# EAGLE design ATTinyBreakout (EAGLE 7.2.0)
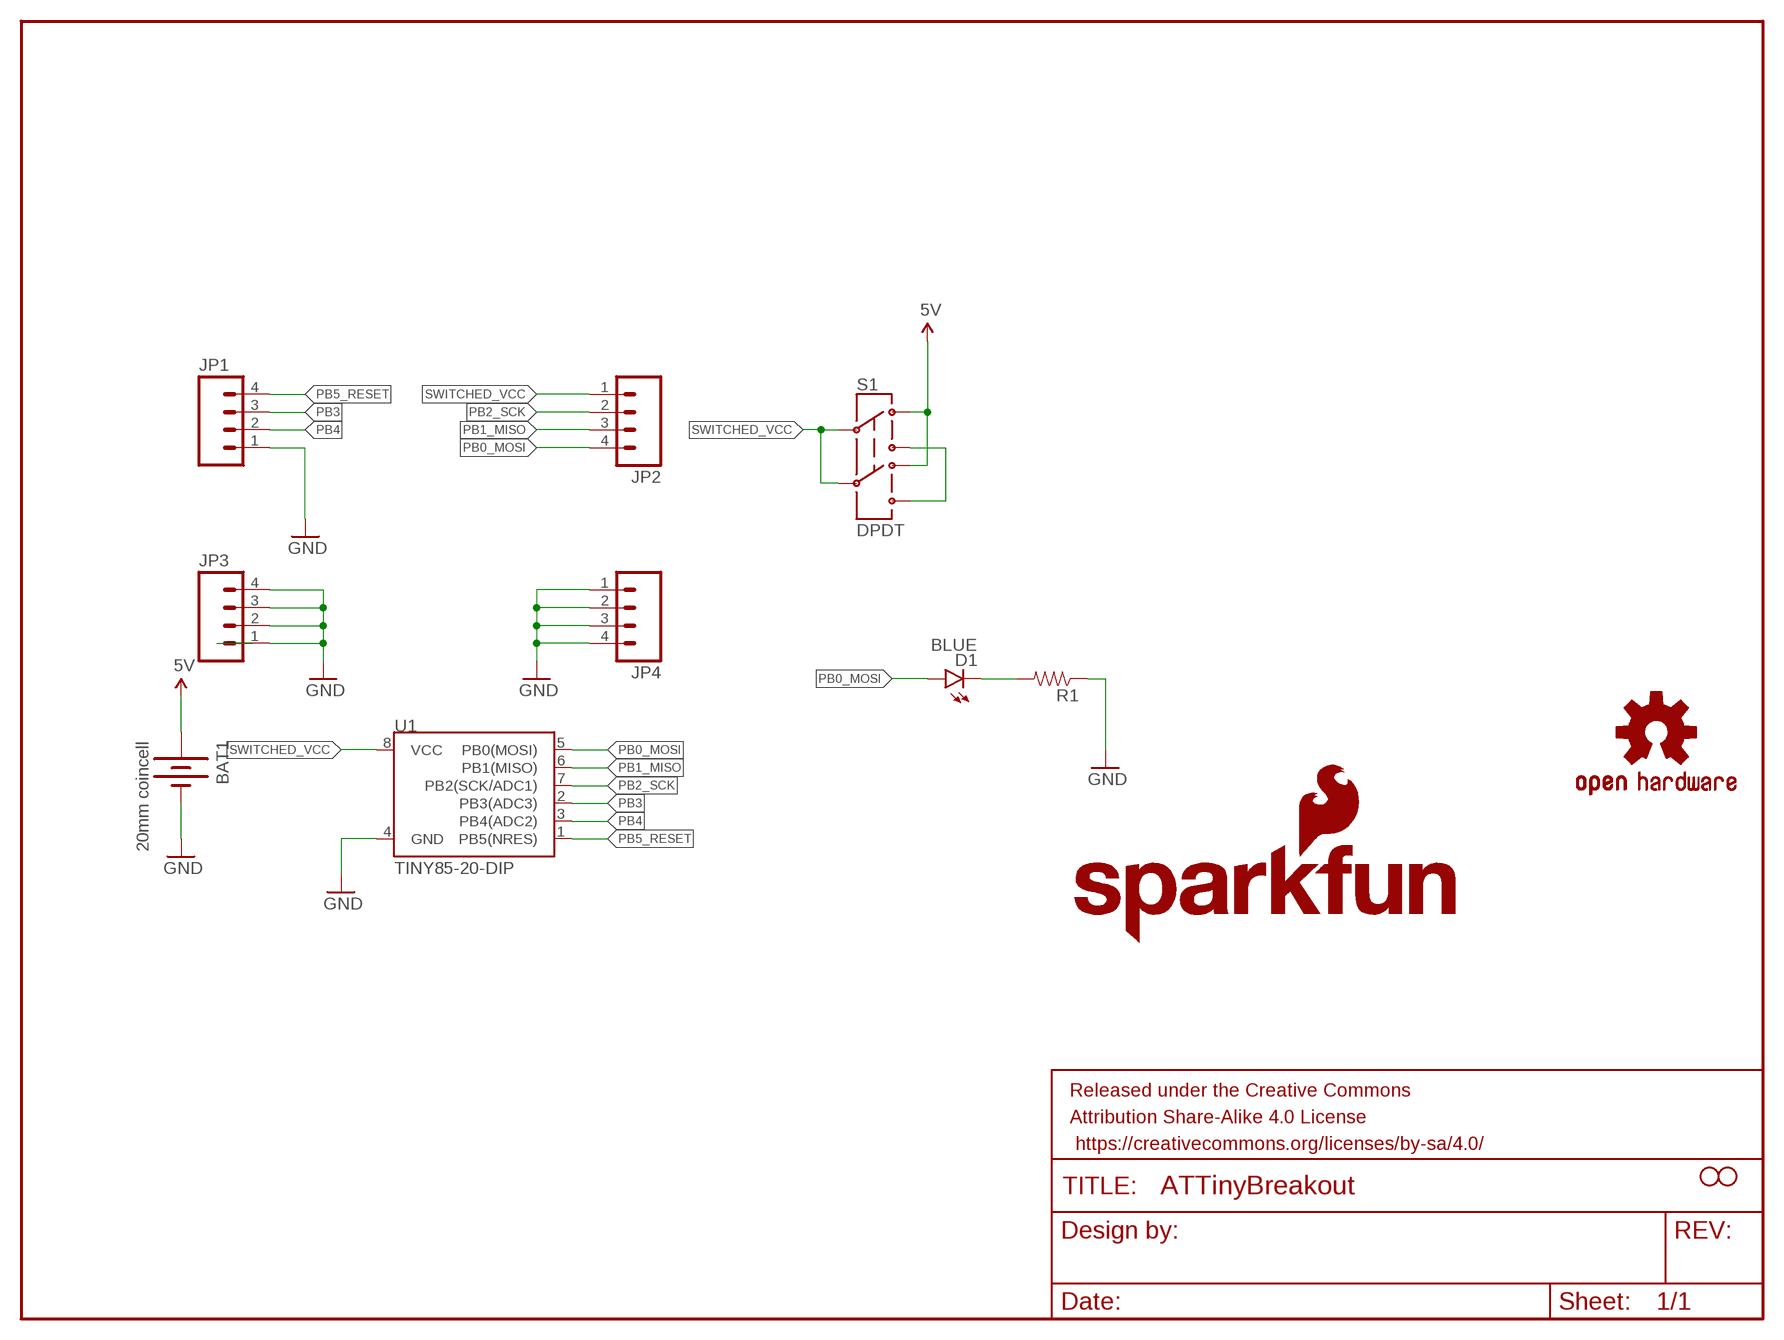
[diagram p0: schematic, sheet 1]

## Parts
BAT1  20mm coincell  BATTERY20MM_4LEGS  [BATTCON_20MM_4LEGS]
D1  BLUE  LED-BLUE0603  [LED-0603]
FRAME1  FRAME-LETTER  [CREATIVE_COMMONS]
JP1  M04LOCK  [1X04_LOCK]
JP2  M04LOCK  [1X04_LOCK]
JP3  M041X04_NO_SILK  [1X04_NO_SILK]
JP4  M041X04_NO_SILK  [1X04_NO_SILK]
LOGO2  SFE_LOGO_FLAME.1_INCH  [SFE_LOGO_FLAME_.1]
LOGO3  OSHW-LOGOS  [OSHW-LOGO-S]
LOGO4  SFE_LOGO_NAME_FLAME.1_INCH  [SFE_LOGO_NAME_FLAME_.1]
R1  RESISTOR0603-RES  [0603-RES]
S1  DPDT  SWITCH-DPDTAYZ0202  [AYZ0202]
STANDOFF1  STAND-OFF  [STAND-OFF]
STANDOFF2  STAND-OFF  [STAND-OFF]
U1  TINY85-20-DIP  ATTINY45TINY85-20-DIP  [DIP08]

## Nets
GND: BAT1.2(-) JP1.1 JP3.1 JP3.2 JP3.3 JP3.4 JP4.1 JP4.2 JP4.3 JP4.4 R1.1 U1.4(GND)
N$1: D1.C R1.2
N$2: S1.3 S1.6
PB0_MOSI: D1.A JP2.4 U1.5(PB0(MOSI))
PB1_MISO: JP2.3 U1.6(PB1(MISO))
PB2_SCK: JP2.2 U1.7(PB2(SCK/ADC1))
PB3: JP1.3 U1.2(PB3(ADC3))
PB4: JP1.2 U1.3(PB4(ADC2))
PB5_RESET: JP1.4 U1.1(PB5(NRES))
SWITCHED_VCC: JP2.1 S1.2 S1.5 U1.8(VCC)
VCC: BAT1.1(+) S1.1 S1.4 ; supply symbol labelled 5V

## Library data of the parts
BAT1 = SparkFun-Electromechanical:BATTERY: Battery Holders; PROD_ID: BATT-10373
D1 = SparkFun-LED:LED-BLUE: Blue LEDs for production use; PROD_ID: DIO-08575
FRAME1 = SparkFun-Aesthetics:FRAME-LETTER: Schematic Frame; DESIGNER: NAME; VERSION: v01
JP1-JP4 = SparkFun-Connectors:M04: Header 4 Standard 4-pin 0.1" header. Use with straight break away headers (SKU : PRT-00116), right angle break away headers (PRT-00553), swiss pins (PRT-00743), machine pins (PRT-00117), and female headers (PRT-00115). Molex polarized connector foot print use with SKU : PRT-08231 with associated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
LOGO2 = SparkFun-Aesthetics:SFE_LOGO_FLAME: SFE Logo, flame only
LOGO3 = SparkFun-Aesthetics:OSHW-LOGO: Open Source Hardware Logo
LOGO4 = SparkFun-Aesthetics:SFE_LOGO_NAME_FLAME: SFE Logo, name and flame
R1 = SparkFun-Passives:RESISTOR: Resistor
S1 = SparkFun-Electromechanical:SWITCH-DPDT: DPDT Version of the COM-00597; PROD_ID: SWCH-08179
STANDOFF1 STANDOFF2 = SparkFun-Electromechanical:STAND-OFF: #4 Stand Off
U1 = SparkFun-DigitalIC:ATTINY45: Atmel 8-pin 2/4/8kB flash uC; PROD_ID: IC-09445

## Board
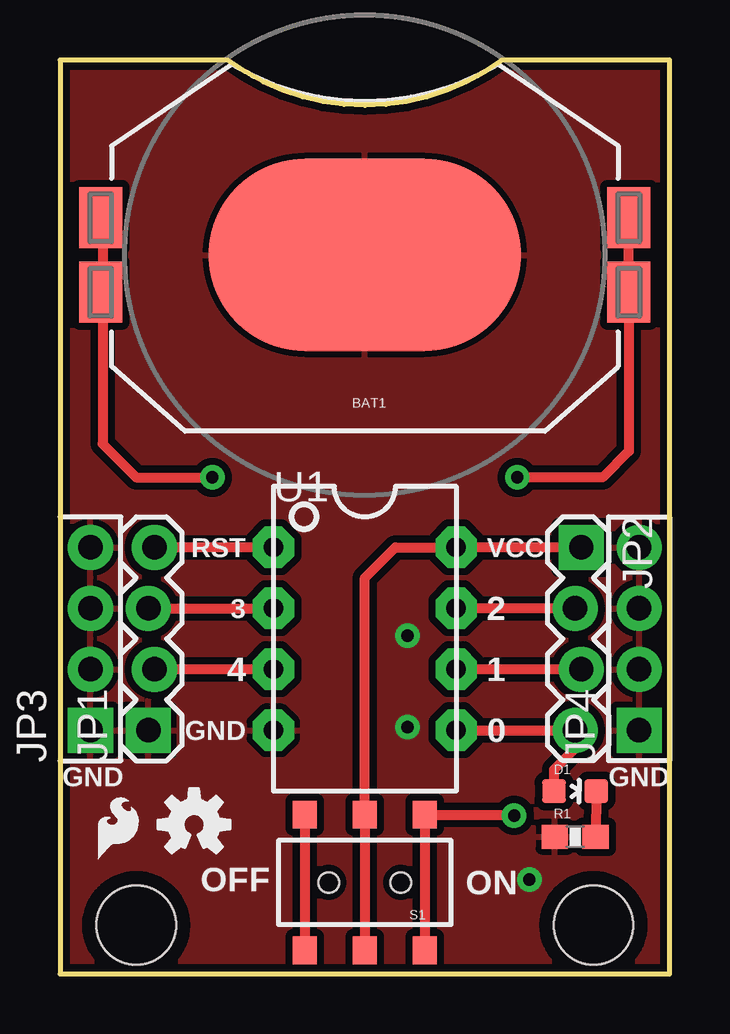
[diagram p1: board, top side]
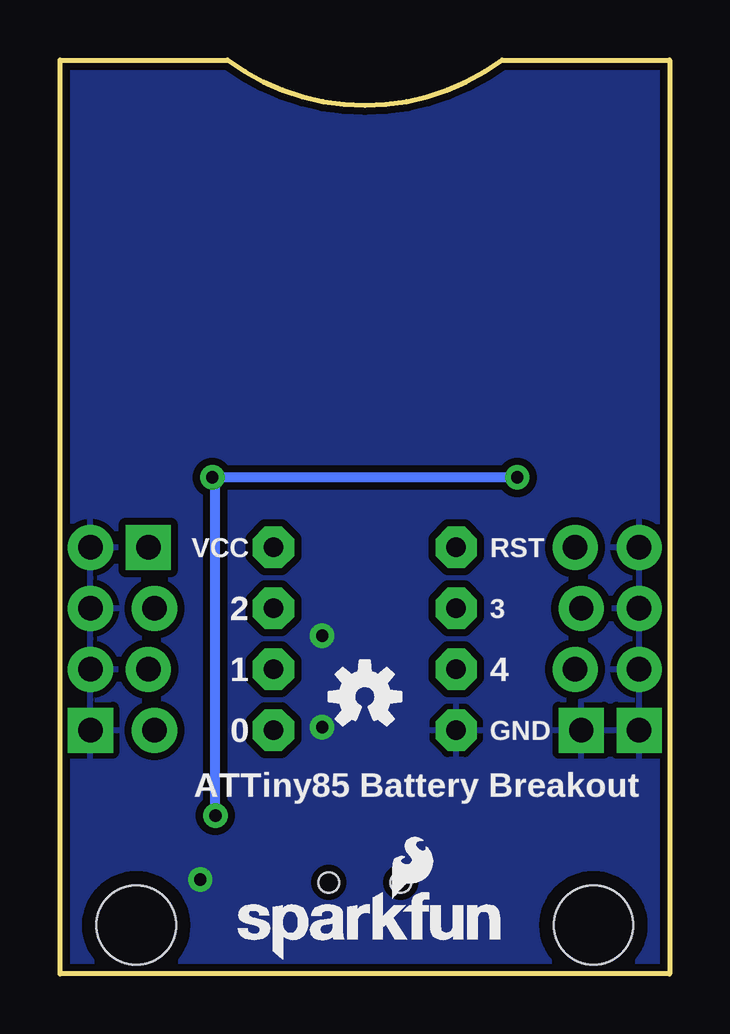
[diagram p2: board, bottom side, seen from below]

Size 25.4 x 38.1 mm. Coordinates in mm from the lower left corner, seen from the top.
Outline: 0,0 25.4,0 25.4,38.1 18.41,38.1 arc-73 6.99,38.1 0,38.1 0,0
Copper layers (1*16): Top 0.035mm / dielectric 1.5mm / Bottom 0.035mm
Design rules "SparkFun-2-layer": minimum track width 7mil, minimum drill 15mil, track to track 8mil, track to pad 8mil, pad to pad 8mil, via to via 8mil, smd to smd 8mil, copper to edge 8mil, drill to drill 8mil, minimum pad ring 12mil, minimum via ring 10mil, stop-mask expansion 4mil, vias tented up to drill 20mil, thermal gap 10mil

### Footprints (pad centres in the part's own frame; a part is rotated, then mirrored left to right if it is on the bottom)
BATTCON_20MM_4LEGS = smd 1.778 x 2.54: 1 -11,1.55; 3 11,1.55; P$1 -11,-1.55; P$2 11,-1.55 | smd 13 x 8: 2 0,0
LED-0603 = smd 1 x 1: A 0,-0.877; C 0,0.877
1X04_LOCK = drill 1.016 pad 1.88 square: 1 0,0.127 | drill 1.016 pad 1.88: 2 2.54,-0.127; 3 5.08,0.127; 4 7.62,-0.127
1X04_NO_SILK = drill 1.016 pad 1.88 square: 1 0,0 | drill 1.016 pad 1.88: 2 2.54,0; 3 5.08,0; 4 7.62,0
0603-RES = smd 1.1 x 1: 1 -0.85,0; 2 0.85,0
AYZ0202 = smd 1 x 1.15: 1 -2.5,2.825; 2 0,2.825; 3 2.5,2.825; 4 -2.5,-2.825; 5 0,-2.825; 6 2.5,-2.825 | hole 0.85: 1.5,0; -1.5,0
STAND-OFF = hole 3.302: 0,0
DIP08 = drill 0.813 pad 1.727 octagon: 1 -3.81,-3.81; 2 -1.27,-3.81; 3 1.27,-3.81; 4 3.81,-3.81; 5 3.81,3.81; 6 1.27,3.81; 7 -1.27,3.81; 8 -3.81,3.81

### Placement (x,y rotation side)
BAT1  12.7,29.97 180 top
D1  21.46,7.62 270 top
FRAME1  not placed on the board
JP1  3.81,10.16 90 top
JP2  21.59,17.78 270 top
JP3  1.27,10.16 90 top
JP4  24.13,10.16 90 top
LOGO2  1.27,4.45 0 top
LOGO3  5.59,6.22 0 top
LOGO4  18.41,0.51 0 bottom
R1  21.46,5.71 0 top
S1  12.7,3.81 180 top
STANDOFF1  22.23,2.03 0 top
STANDOFF2  3.17,2.03 0 top
U1  12.7,13.97 270 top
U$1  OSHW-LOGOS  [OSHW-LOGO-S]  12.7,11.56 0 bottom

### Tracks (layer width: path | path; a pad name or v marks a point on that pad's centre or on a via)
GND  (via drill 0.51)
  other vias: 19.56,3.94 14.48,14.1 14.48,10.29
  pour Bottom (isolate 0.305): 0,38.1 25.4,38.1 25.4,0 0,0
  pour Top (isolate 0.305): 0,0 25.4,0 25.4,38.1 0,38.1
N$1
  Top 0.406: D1.C R1.2
N$2
  Top 0.406: S1.6 S1.3
PB0_MOSI
  Top 0.406: U1.5 JP2.4 21.46,9.4 20.59,8.52 D1.A
PB1_MISO
  Top 0.406: JP2.3 U1.6
PB2_SCK
  Top 0.406: JP2.2 U1.7 JP2.2
PB3
  Top 0.406: JP1.3 U1.2
PB4
  Top 0.406: U1.3 JP1.2
PB5_RESET
  Top 0.406: U1.1 JP1.4
SWITCHED_VCC
  Top 0.406: S1.2 S1.5 12.7,16.51 13.97,17.78 U1.8 JP2.1
VCC  (via drill 0.51)
  Top 0.406: 1.65,31.37 1.78,31.24 1.78,22.1 3.17,20.7 v6.35,20.7 | 23.62,32 23.7,31.93 BAT1.1 23.7,21.8 22.61,20.7 v19.05,20.7 | S1.1 S1.4 18.89,6.63 v18.92,6.6
  Bottom 0.406: v18.92,6.6 18.92,20.57 v19.05,20.7 v6.35,20.7

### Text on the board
tPlace: RST | VCC | 3 | 2 | 4 | 1 | GND | 0 | GND | GND | OFF | ON
bPlace: RST | VCC | 3 | 2 | 4 | 1 | GND | 0 | ATTiny85 Battery Breakout
tDocu: Brian Huang

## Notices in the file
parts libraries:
SparkFun-Aesthetics: Licensing: Creative Commons ShareAlike 4.0 International - https://creativecommons.org/licenses/by-sa/4.0
SparkFun-Aesthetics: Released under the Creative Commons Attribution Share-Alike 4.0 License
SparkFun-Aesthetics: https://creativecommons.org/licenses/by-sa/4.0
